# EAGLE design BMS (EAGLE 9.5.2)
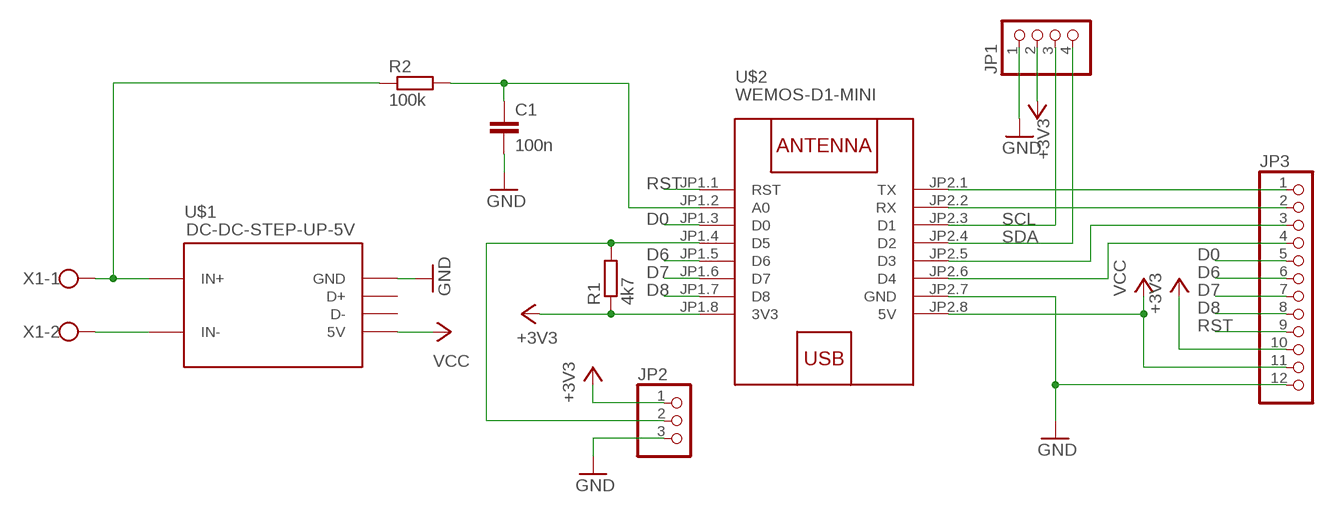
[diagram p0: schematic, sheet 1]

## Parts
C1  100n  C-EUC0603  [C0603]
JP1  PINHD-1X4  [1X04]
JP2  PINHD-1X3  [1X03]
JP3  PINHD-1X12  [1X12]
R1  4k7  R-EU_R0603  [R0603]
R2  100k  R-EU_R0603  [R0603]
U$1  DC-DC-STEP-UP-5V  [DC-DC-STEP-UP-5V]
U$2  WEMOS-D1-MINI  [WEMOS-D1-MINI]
X1  W237-102  [W237-102]

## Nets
+3V3: JP1.2 JP2.1 JP3.10 R1.1 U$2.JP1.8(3V3)
D0: JP3.5 U$2.JP1.3(D0)
D3: JP3.3 U$2.JP2.5(D3)
D4: JP3.4 U$2.JP2.6(D4)
D6: JP3.6 U$2.JP1.5(D6)
D7: JP3.7 U$2.JP1.6(D7)
D8: JP3.8 U$2.JP1.7(D8)
GND: C1.2 JP1.1 JP2.3 JP3.12 U$1.GND U$2.JP2.7(GND)
N$1: R2.1 U$1.IN+ X1.1
N$2: U$1.IN- X1.2
N$5: JP2.2 R1.2 U$2.JP1.4(D5)
N$7: C1.1 R2.2 U$2.JP1.2(A0)
RST: JP3.9 U$2.JP1.1(RST)
RX: JP3.2 U$2.JP2.2(RX)
SCL: JP1.3 U$2.JP2.3(D1)
SDA: JP1.4 U$2.JP2.4(D2)
TX: JP3.1 U$2.JP2.1(TX)
VCC: JP3.11 U$1.5V U$2.JP2.8(5V)
Unconnected: U$1.D+ U$1.D-

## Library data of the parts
C1 = rcl:C-EU: CAPACITOR, European symbol; SPICEPREFIX: C
JP1 = pinhead:PINHD-1X4: PIN HEADER
JP2 = pinhead:PINHD-1X3: PIN HEADER
JP3 = pinhead:PINHD-1X12: PIN HEADER
R1 R2 = rcl:R-EU_: RESISTOR, European symbol; SPICEPREFIX: R
U$1 = diy-modules:DC-DC-STEP-UP-5V: DC/DC Step-Up Converter
U$2 = diy-modules:WEMOS-D1-MINI: WEMOS D1 mini: Mini Wi-Fi Board based on ESP-8266 device More details can be found here: https://www.wemos.cc/product/d1-mini.html Click here to find device on ebay.com
X1 = con-wago-500:W237-102: WAGO SCREW CLAMP; MPN: 237-102; OC_FARNELL: unknown; OC_NEWARK: 70K9898

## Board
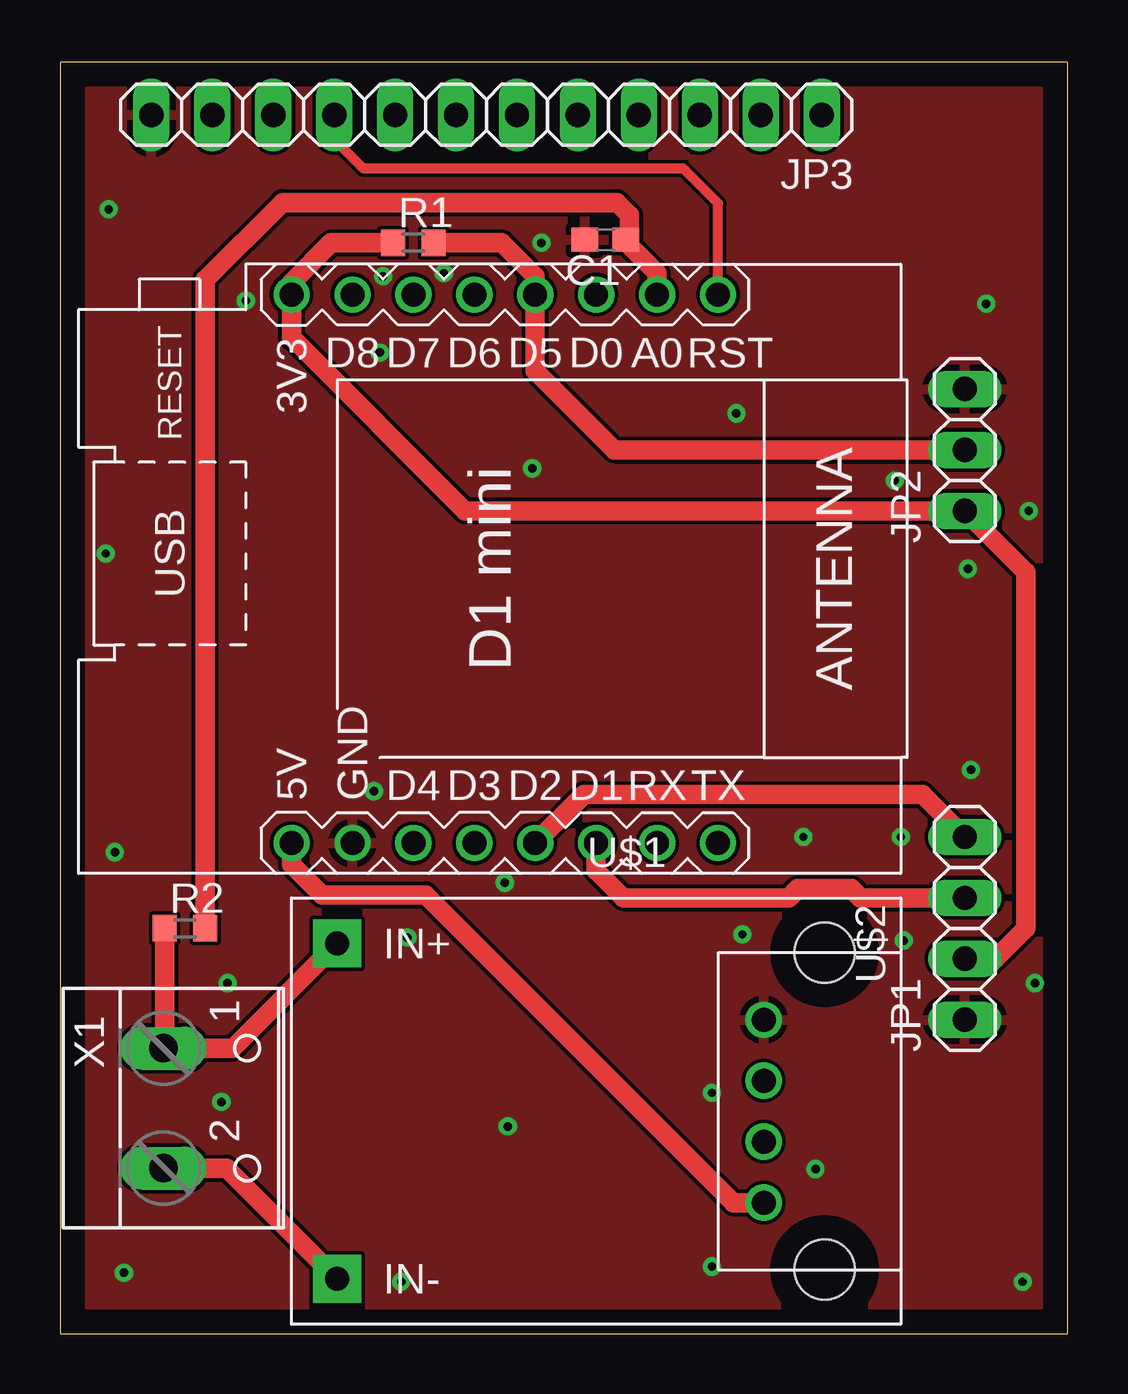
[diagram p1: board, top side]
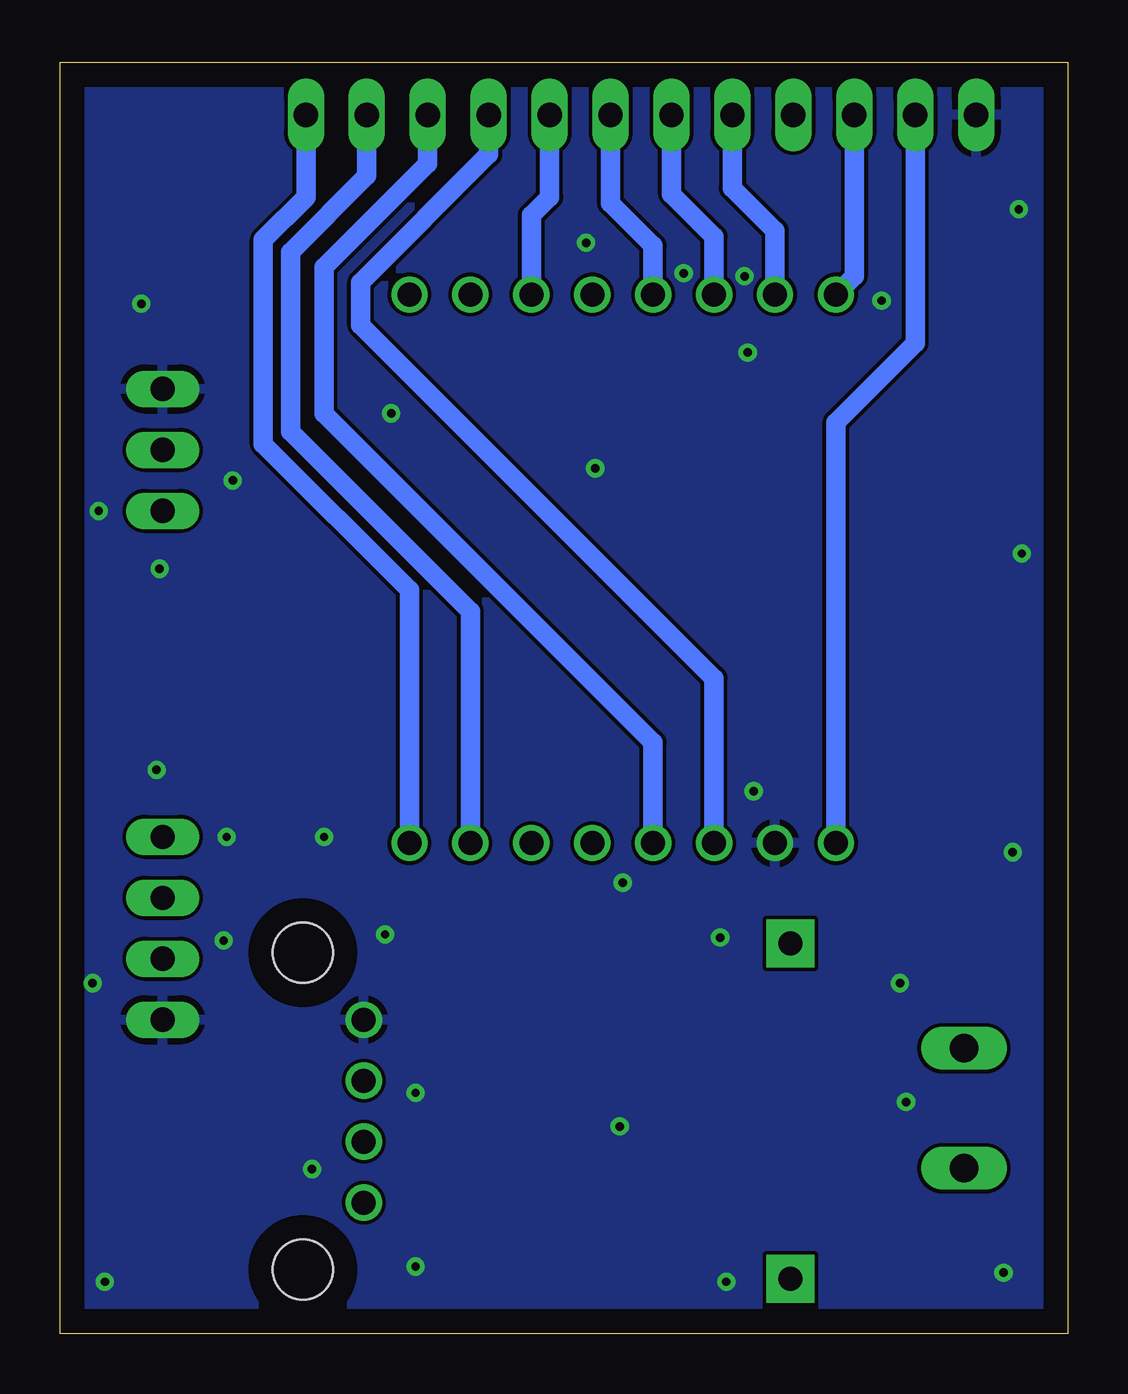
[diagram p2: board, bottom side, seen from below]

Size 42 x 53 mm. Coordinates in mm from the lower left corner, seen from the top.
Outline: 0,0 42,0 42,53 0,53 0,0
Copper layers (1*16): Top 0.035mm / dielectric 0.15mm / Bottom 0.035mm
Design rules "default": minimum track width 6mil, minimum drill 0.35mm, track to track 6mil, track to pad 6mil, pad to pad 6mil, via to via 6mil, smd to smd 6mil, copper to edge 40mil, drill to drill 6mil, minimum pad ring 10mil, minimum via ring 8mil, stop-mask expansion 4mil, vias tented up to drill 0mil, thermal gap 10mil

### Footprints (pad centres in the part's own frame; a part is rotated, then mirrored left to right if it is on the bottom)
C0603 = smd 1.1 x 1: 1 -0.85,0; 2 0.85,0
1X04 = drill 1.016 long: 1 -3.81,0; 2 -1.27,0; 3 1.27,0; 4 3.81,0
1X03 = drill 1.016 long: 1 -2.54,0; 2 0,0; 3 2.54,0
1X12 = drill 1.016 long: 1 -13.97,0; 2 -11.43,0; 3 -8.89,0; 4 -6.35,0; 5 -3.81,0; 6 -1.27,0; 7 1.27,0; 8 3.81,0; 9 6.35,0; 10 8.89,0; 11 11.43,0; 12 13.97,0
R0603 = smd 1 x 1.1: 1 -0.85,0; 2 0.85,0
DC-DC-STEP-UP-5V = drill 1: 5V 6.985,-3.81; D+ 6.985,1.27; D- 6.985,-1.27; GND 6.985,3.81 | drill 1 pad 2 square: IN+ -10.795,6.985; IN- -10.795,-6.985 | hole 2.5: 9.525,6.604; 9.525,-6.604
WEMOS-D1-MINI = drill 1: JP1.1 -11.43,9.525; JP1.2 -11.43,6.985; JP1.3 -11.43,4.445; JP1.4 -11.43,1.905; JP1.5 -11.43,-0.635; JP1.6 -11.43,-3.175; JP1.7 -11.43,-5.715; JP1.8 -11.43,-8.255; JP2.1 11.43,9.525; JP2.2 11.43,6.985; JP2.3 11.43,4.445; JP2.4 11.43,1.905; JP2.5 11.43,-0.635; JP2.6 11.43,-3.175; JP2.7 11.43,-5.715; JP2.8 11.43,-8.255
W237-102 = drill 1.194 long: 1 -2.5,-1.27; 2 2.5,-1.27

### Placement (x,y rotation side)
C1  22.73,45.59 180 top
JP1  37.72,16.89 90 top
JP2  37.72,36.83 90 top
JP3  17.78,50.8 180 top
R1  14.73,45.47 0 top
R2  5.21,16.89 0 top
U$1  22.35,9.27 0 top
U$2  17.91,31.88 270 top
X1  5.59,9.4 270 top

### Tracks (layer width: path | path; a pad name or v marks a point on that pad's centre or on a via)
+3V3
  Top 0.813: JP1.2 38.99,15.62 40.26,16.89 40.26,31.75 JP2.1 16.89,34.29 9.65,41.53 U$2.JP1.8 9.65,43.81 11.3,45.47 R1.1
  Bottom 0.813: JP3.10 8.89,44.07 U$2.JP1.8
D0
  Bottom 0.813: U$2.JP1.3 22.35,46.61 21.59,47.37 JP3.5
D3
  Bottom 0.813: U$2.JP2.5 17.27,24.64 30.99,38.35 30.99,44.45 26.67,48.77 JP3.3
D4
  Bottom 0.813: U$2.JP2.6 14.73,27.3 29.46,42.04 29.46,43.81 24.13,49.15 JP3.4
D6
  Bottom 0.813: U$2.JP1.5 17.27,45.34 19.05,47.12 JP3.6
D7
  Bottom 0.813: U$2.JP1.6 14.73,45.72 16.51,47.5 JP3.7
D8
  Bottom 0.813: JP3.8 13.97,47.75 12.19,45.97 U$2.JP1.7
GND  (via drill 0.35)
  other vias: 19.68,36.07 13.34,40.89 20.07,45.47 13.46,44.07 16,44.2 7.75,43.05 37.97,23.5 40.39,34.29 6.99,14.61 14.48,16.51 6.73,9.65 27.18,2.79 2.67,2.54 2.29,20.07 40.13,2.16 40.64,14.61 31.5,6.86 1.91,32.51 2.03,46.86 38.61,42.93 28.19,38.35 34.8,35.56 37.85,31.88 30.99,20.7 35.05,20.7 18.54,18.8 13.08,22.61 14.22,2.16 18.67,8.64 27.18,10.03 28.45,16.64 35.18,16.38
  pour Top: -2.54,-1.27 -2.54,58.42 45.72,58.42 45.72,-1.27
  pour Bottom: -3.81,55.88 -3.81,-3.81 46.99,-3.81 46.99,55.88
N$1
  Top 0.813: U$1.IN+ 7.2,11.9 X1.1 4.36,11.94 R2.1
N$2
  Top 0.813: X1.2 6.95,6.9 U$1.IN-
N$5
  Top 0.813: R1.2 18.41,45.47 19.81,44.07 U$2.JP1.4 19.81,40.13 23.11,36.83 JP2.2
N$7
  Top 0.813: U$2.JP1.2 24.89,44.2 23.58,45.51 C1.1 23.75,45.76 23.75,46.61 23.21,47.14 9.27,47.14 6.06,43.93 R2.2
RST
  Top 0.406: U$2.JP1.1 27.43,47.12 25.99,48.56 12.65,48.56 11.43,49.78 JP3.9
RX
  Bottom 0.813: U$2.JP2.2 24.89,30.1 32.38,37.59 32.38,45.09 29.21,48.26 JP3.2
SCL
  Top 0.813: U$2.JP2.3 22.35,19.3 23.5,18.16 30.38,18.16 30.77,18.55 32.98,18.55 33.37,18.16 JP1.3
SDA
  Top 0.813: U$2.JP2.4 21.84,22.48 35.94,22.48 JP1.4
TX
  Bottom 0.813: U$2.JP2.1 27.43,30.99 33.53,37.08 33.53,45.59 31.75,47.37 JP3.1
VCC
  Top 0.813: U$2.JP2.8 9.65,19.56 10.92,18.29 15.24,18.29 28.07,5.46 U$1.5V
  Bottom 0.813: U$2.JP2.8 9.65,37.97 6.35,41.27 JP3.11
